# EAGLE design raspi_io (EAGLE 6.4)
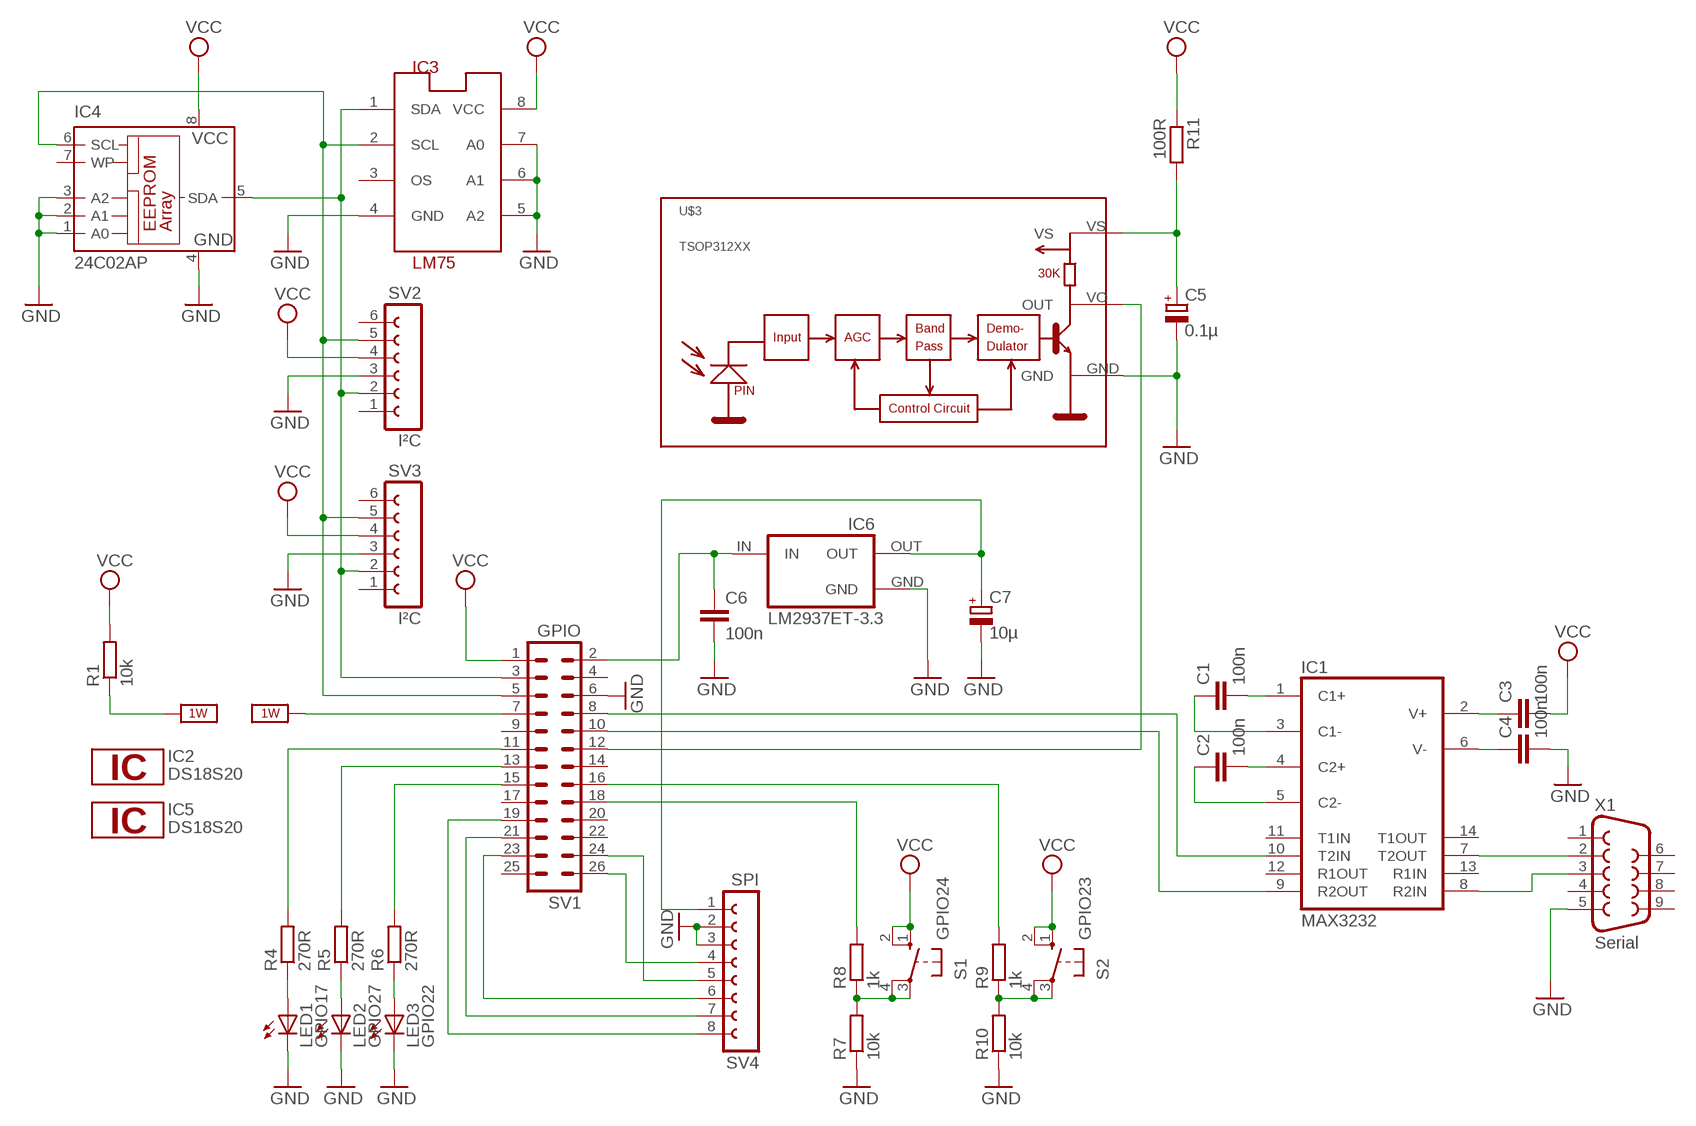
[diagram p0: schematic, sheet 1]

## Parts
C1  100n  C-EU025-025X050  [C025-025X050]
C2  100n  C-EU025-025X050  [C025-025X050]
C3  100n  C-EU025-025X050  [C025-025X050]
C4  100n  C-EU025-025X050  [C025-025X050]
C5  0.1µ  CPOL-EUE2-5  [E2-5]
C6  100n  C-EU025-025X050  [C025-025X050]
C7  10µ  CPOL-EUE2-5  [E2-5]
IC1  MAX3232  MAX232  [DIL16]
IC2  DS18S20  [TO92-]
IC3  LM75  LM75_ICN  [SO8_LM75]
IC4  24C02AP  [DIL8]
IC5  DS18S20  [TO92-]
IC6  LM2937ET-3.3  [TO220(V)]
LED1  GPIO17  LED3MM  [LED3MM]
LED2  GPIO27  LED3MM  [LED3MM]
LED3  GPIO22  LED3MM  [LED3MM]
R1  10k  R-EU_0207/10  [0207/10]
R4  270R  R-EU_0207/10  [0207/10]
R5  270R  R-EU_0207/10  [0207/10]
R6  270R  R-EU_0207/10  [0207/10]
R7  10k  R-EU_0207/10  [0207/10]
R8  1k  R-EU_0207/10  [0207/10]
R9  1k  R-EU_0207/10  [0207/10]
R10  10k  R-EU_0207/10  [0207/10]
R11  100R  R-EU_0207/10  [0207/10]
S1  GPIO24  10-XX  [B3F-10XX]
S2  GPIO23  10-XX  [B3F-10XX]
SV1  GPIO  ML26  [ML26]
SV2  I²C  FE06-1  [FE06]
SV3  I²C  FE06-1  [FE06]
SV4  SPI  FE08-1  [FE08]
U$3  TSOP312XX  [TSOP312]
X1  Serial  F09HP  [F09HP]

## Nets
1W: R1.1 SV1.7 ; supply symbol labelled 1W_SUP
GND: C4.2 C5.- C6.2 C7.- IC3.4(GND) IC3.5(A2) IC3.6(A1) IC3.7(A0) IC4.1(A0) IC4.2(A1) IC4.3(A2) IC4.4(GND) IC6.GND LED1.K(C) LED2.K(C) LED3.K(C) R7.1 R10.1 SV1.6 SV2.3 SV3.3 SV4.2 SV4.3 U$3.GND X1.5
N$1: C1.2 IC1.1(C1+)
N$2: C1.1 IC1.3(C1-)
N$3: C2.2 IC1.4(C2+)
N$4: C2.1 IC1.5(C2-)
N$5: C3.1 IC1.2(V+)
N$6: C4.1 IC1.6(V-)
N$7: IC1.10(T2IN) SV1.8
N$8: IC1.9(R2OUT) SV1.10
N$9: IC1.7(T2OUT) X1.2
N$10: IC1.8(R2IN) X1.3
N$11: IC3.1(SDA) IC4.5(SDA) SV1.3 SV2.2 SV3.2
N$12: IC3.2(SCL) IC4.6(SCL) SV1.5 SV2.5 SV3.5
N$13: LED1.A R4.1
N$14: LED2.A R5.1
N$15: LED3.A R6.1
N$16: R4.2 SV1.11
N$17: R5.2 SV1.13
N$18: R6.2 SV1.15
N$19: R7.2 R8.1 S1.3(P) S1.4(P1)
N$21: R8.2 SV1.18
N$22: R9.2 SV1.16
N$23: C5.+ R11.2 U$3.VS
N$24: SV1.12 U$3.VO(OUT)
N$25: R9.1 R10.2 S2.3(P) S2.4(P1)
N$26: SV1.19 SV4.8
N$27: SV1.21 SV4.7
N$28: SV1.23 SV4.6
N$29: SV1.24 SV4.5
N$30: SV1.26 SV4.4
N$32: C6.1 IC6.IN SV1.2
N$33: C7.+ IC6.OUT SV4.1
VCC: C3.2 IC3.8(VCC) IC4.8(VCC) R1.2 R11.1 S1.1(S) S1.2(S1) S2.1(S) S2.2(S1) SV1.1 SV2.4 SV3.4
Unconnected: IC1.11(T1IN) IC1.12(R1OUT) IC1.13(R1IN) IC1.14(T1OUT) IC3.3(OS) IC4.7(WP) SV1.4 SV1.9 SV1.14 SV1.17 SV1.20 SV1.22 SV1.25 SV2.1 SV2.6 SV3.1 SV3.6 X1.1 X1.4 X1.6 X1.7 X1.8 X1.9

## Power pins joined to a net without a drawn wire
1W: IC2.2 IC5.2
GND: IC1.15(GND) IC2.1 IC5.1
VCC: IC1.16(VCC) IC2.3 IC5.3

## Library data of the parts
C1-C4 C6 = rcl:C-EU: CAPACITOR, European symbol
C5 C7 = rcl:CPOL-EU: POLARIZED CAPACITOR, European symbol
IC1 = maxim:MAX232: RS232 TRANSEIVER; MF: MAXIM; MPN: MAX232ACPE+; OC_FARNELL: 9723773; OC_NEWARK: 68K4544
IC2 IC5 = 1wire:DS18S20: High Precision Digital Thermometer This chip provides a onewire thermosensor with approx. 0.5°C accuracy.A programmable over/undertemperure alarm is available. Notes: Vdd must be applied for accurate measurements at low temperatures, as the parasite power circuit otherwise heats the sensor. If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
IC3 = lm75:LM75_IC: Temperatursensor
IC4 = microchip:24*: Serial EEPROM I2C; MF: MICROCHIP; MPN: 24C02C-I/P; OC_FARNELL: 1755843; OC_NEWARK: 96K4062
IC6 = lm2937:LM2937ET*: 400 and 500 mA Low Dropout Voltage Regulator NATIONAL SEMICONDUCTOR created by Peter.Hofmann@ph-tronic.de 10-2004 Rev.0
LED1-LED3 = led:LED: LED
R1 R4-R11 = rcl:R-EU_: RESISTOR, European symbol
S1 S2 = switch-omron:10-XX: OMRON SWITCH; MPN: B3F-1000; OC_FARNELL: 176432; OC_NEWARK: 36M3542
SV1 = con-harting-ml:ML26: HARTING; OC_FARNELL: unknown; OC_NEWARK: unknown
SV2 SV3 = con-lsta:FE06-1: FEMALE HEADER; OC_FARNELL: unknown; OC_NEWARK: unknown
SV4 = con-lsta:FE08-1: FEMALE HEADER; OC_FARNELL: unknown; OC_NEWARK: unknown
U$3 = vishay:TSOP312XX
X1 = con-subd:F09: SUB-D; OC_FARNELL: unknown; OC_NEWARK: unknown

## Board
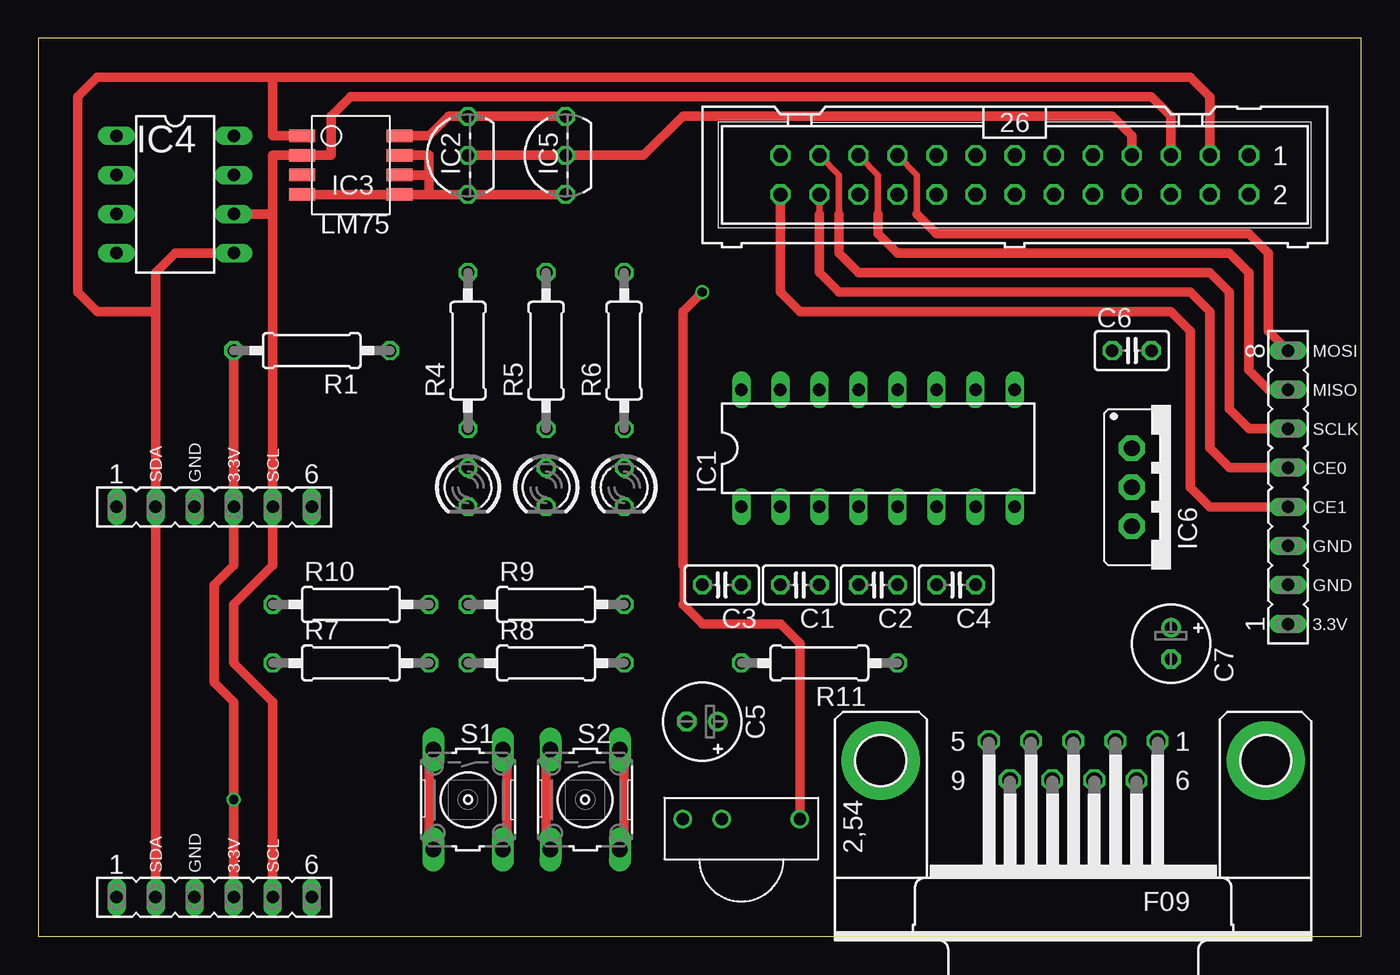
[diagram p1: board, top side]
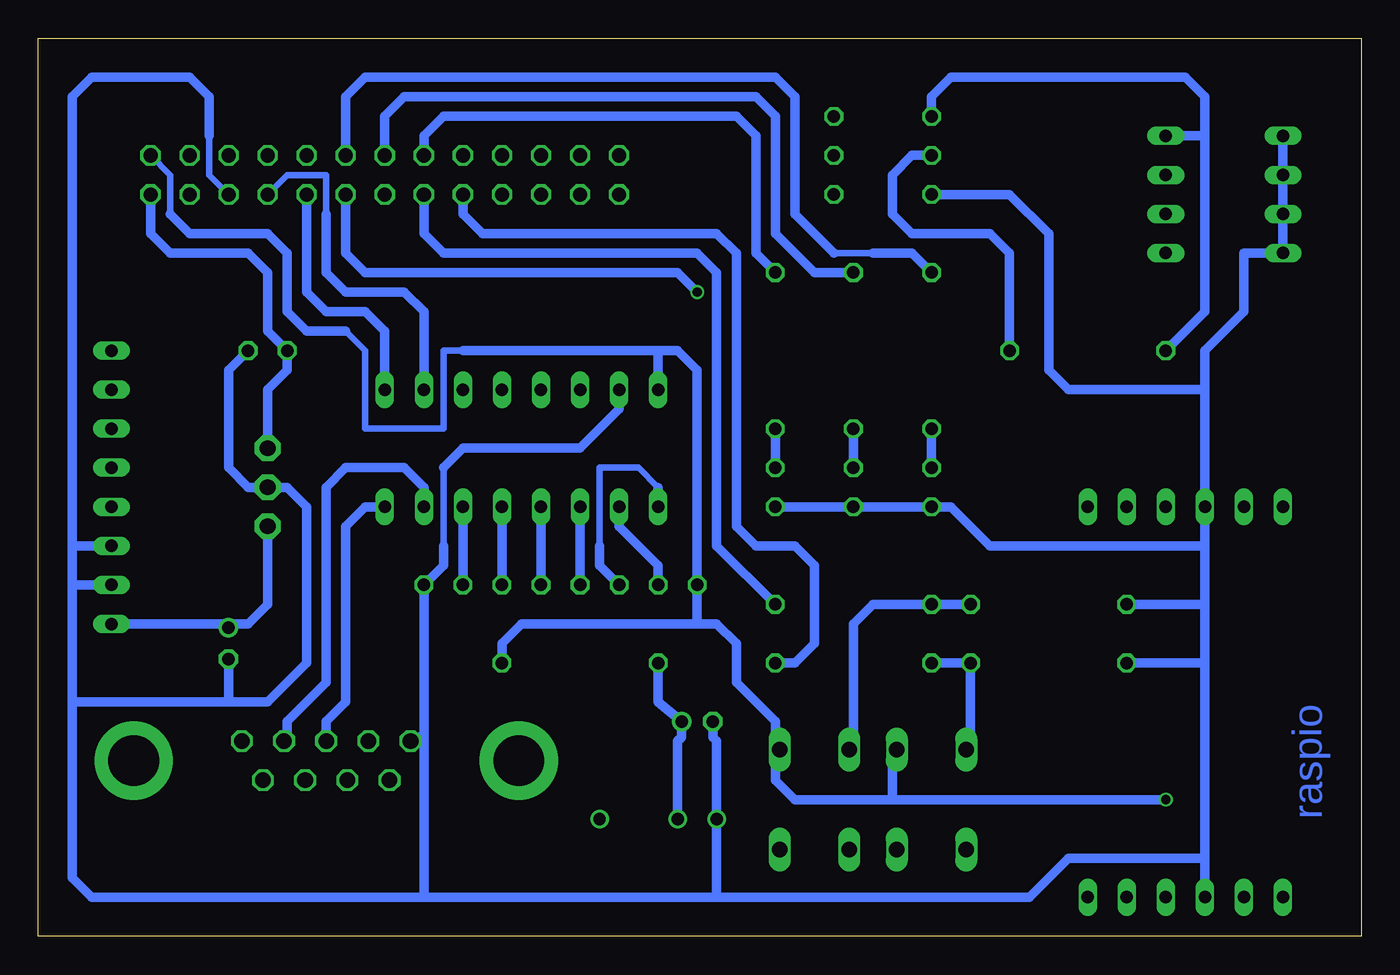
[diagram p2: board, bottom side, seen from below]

Size 86.03 x 58.41 mm. Coordinates in mm from the lower left corner, seen from the top.
Outline: 0,0 86.03,0 86.03,58.41 0,58.41 0,0
Copper layers (1*16): Top 0.035mm / dielectric 1.5mm / Bottom 0.035mm
Design rules "PCB-POOL Standard": minimum track width 0.15mm, minimum drill 0.3mm, track to track 0.15mm, track to pad 0.15mm, pad to pad 0.15mm, via to via 0.15mm, smd to smd 0.15mm, copper to edge 0.3mm, drill to drill 0.2mm, minimum pad ring 0.2mm, minimum via ring 0.15mm, stop-mask expansion 0.075mm, vias tented up to drill 0mil, thermal gap 0.2mm

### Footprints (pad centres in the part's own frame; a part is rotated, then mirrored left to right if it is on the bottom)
C025-025X050 = drill 0.813 octagon: 1 -1.27,0; 2 1.27,0
E2-5 = drill 0.813 pad 1.27: + -1.016,0 | drill 0.813 pad 1.27 octagon: - 1.016,0
DIL16 = drill 0.813 long: 1 -8.89,-3.81; 2 -6.35,-3.81; 3 -3.81,-3.81; 4 -1.27,-3.81; 5 1.27,-3.81; 6 3.81,-3.81; 7 6.35,-3.81; 8 8.89,-3.81; 9 8.89,3.81; 10 6.35,3.81; 11 3.81,3.81; 12 1.27,3.81; 13 -1.27,3.81; 14 -3.81,3.81; 15 -6.35,3.81; 16 -8.89,3.81
TO92- = drill 0.813 octagon: 1 -2.54,0; 2 0,0; 3 2.54,0
SO8_LM75 = smd 0.813 x 1.676: 1 -1.27,-3.175; 2 0,-3.175; 3 1.27,-3.175; 4 2.54,-3.175; 5 2.54,3.175; 6 1.27,3.175; 7 0,3.175; 8 -1.27,3.175
DIL8 = drill 0.813 long: 1 -3.81,-3.81; 2 -1.27,-3.81; 3 1.27,-3.81; 4 3.81,-3.81; 5 3.81,3.81; 6 1.27,3.81; 7 -1.27,3.81; 8 -3.81,3.81
TO220(V) = drill 1.016 pad 1.676 octagon: GND 0,0; IN -2.54,0; OUT 2.54,0
LED3MM = drill 0.813 octagon: A -1.27,0; K 1.27,0
0207/10 = drill 0.813 octagon: 1 -5.08,0; 2 5.08,0
B3F-10XX = drill 1.016 long: 1 -3.251,2.261; 2 3.251,2.261; 3 -3.251,-2.261; 4 3.251,-2.261
ML26 = drill 0.914 octagon: 1 -15.24,-1.27; 2 -15.24,1.27; 3 -12.7,-1.27; 4 -12.7,1.27; 5 -10.16,-1.27; 6 -10.16,1.27; 7 -7.62,-1.27; 8 -7.62,1.27; 9 -5.08,-1.27; 10 -5.08,1.27; 11 -2.54,-1.27; 12 -2.54,1.27; 13 0,-1.27; 14 0,1.27; 15 2.54,-1.27; 16 2.54,1.27; 17 5.08,-1.27; 18 5.08,1.27; 19 7.62,-1.27; 20 7.62,1.27; 21 10.16,-1.27; 22 10.16,1.27; 23 12.7,-1.27; 24 12.7,1.27; 25 15.24,-1.27; 26 15.24,1.27
FE06 = drill 0.813 long: 1 -6.35,0; 2 -3.81,0; 3 -1.27,0; 4 1.27,0; 5 3.81,0; 6 6.35,0
FE08 = drill 0.813 long: 1 -8.89,0; 2 -6.35,0; 3 -3.81,0; 4 -1.27,0; 5 1.27,0; 6 3.81,0; 7 6.35,0; 8 8.89,0
TSOP312 = drill 0.8: GND -3.81,0; VO 3.81,0; VS -1.27,0
F09HP = drill 1.016 octagon: 1 -5.486,-1.27; 2 -2.743,-1.27; 3 0,-1.27; 4 2.743,-1.27; 5 5.486,-1.27; 6 -4.115,1.27; 7 -1.372,1.27; 8 1.372,1.27; 9 4.115,1.27 | drill 3.302 pad 5.08: G1 -12.522,0; G2 12.522,0

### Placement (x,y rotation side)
C1  49.53,22.86 180 top
C2  54.61,22.86 180 top
C3  44.45,22.86 180 top
C4  59.69,22.86 0 top
C5  43.18,13.97 180 top
C6  71.12,38.1 0 top
C7  73.66,19.05 270 top
IC1  54.61,31.75 0 top
IC2  27.94,50.8 90 top
IC3  20.32,50.8 270 top
IC4  8.89,48.26 270 top
IC5  34.29,50.8 90 top
IC6  71.12,29.21 270 top
LED1  27.94,29.21 270 top
LED2  33.02,29.21 270 top
LED3  38.1,29.21 270 top
R1  17.78,38.1 180 top
R4  27.94,38.1 90 top
R5  33.02,38.1 90 top
R6  38.1,38.1 90 top
R7  20.32,17.78 0 top
R8  33.02,17.78 0 top
R9  33.02,21.59 0 top
R10  20.32,21.59 0 top
R11  50.8,17.78 180 top
S1  27.94,8.89 270 top
S2  35.56,8.89 270 top
SV1  63.5,49.53 180 top
SV2  11.43,27.94 0 top
SV3  11.43,2.54 0 top
SV4  81.28,29.21 90 top
U$3  45.72,7.62 0 top
X1  67.31,11.43 180 top

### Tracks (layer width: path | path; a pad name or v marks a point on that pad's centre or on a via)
1W
  Top 0.61: IC2.2 IC5.2 39.37,50.8 41.91,53.34 69.85,53.34 71.12,52.07 SV1.7
  Bottom 0.61: IC2.2 29.21,50.8 30.48,49.53 30.48,46.99 29.21,45.72 24.13,45.72 22.86,44.45 R1.1
GND
  Top 0.61: IC3.7 25.4,50.8 25.4,49.53 | 25.4,49.53 25.4,48.26 | 25.4,48.26 IC2.1 IC5.1 | IC3.4 IC3.5 25.4,48.26 | IC3.6 25.4,49.53
  Bottom 0.406: SV1.6 74.93,49.53 74.93,52.07 | 59.69,30.48 59.69,25.4
  Bottom 0.61: LED3.K LED2.K LED1.K 26.67,27.94 24.13,25.4 10.16,25.4 | IC4.1 IC4.2 IC4.3 IC4.4 7.62,44.45 7.62,40.64 10.16,38.1 10.16,35.56 | 74.93,52.07 74.93,54.61 76.2,55.88 82.55,55.88 83.82,54.61 83.82,25.4 | 83.82,25.4 83.82,22.86 | 83.82,22.86 83.82,15.24 | 83.82,15.24 83.82,3.81 82.55,2.54 60.96,2.54 | 60.96,2.54 60.96,13.11 | 41.91,2.54 60.96,2.54 | 41.91,2.54 U$3.GND 41.91,12.7 42.16,12.95 C5.- | 41.91,2.54 21.59,2.54 19.05,5.08 10.16,5.08 | 12.7,17.78 R7.1 10.16,17.78 | 60.96,13.11 C4.2 59.69,24.13 59.69,25.4 | 60.96,13.11 X1.5 | IC1.15 48.26,34.29 50.8,31.75 58.42,31.75 59.69,30.48 | 73.66,15.24 71.12,15.24 68.58,17.78 68.58,27.94 69.85,29.21 IC6.GND 72.39,29.21 73.66,30.48 73.66,36.83 C6.2 | 73.66,15.24 83.82,15.24 | SV4.2 83.82,22.86 | SV4.3 83.82,25.4 | C7.- 73.66,15.24 | 10.16,35.56 SV2.3 10.16,25.4 | 10.16,25.4 10.16,21.59 | 10.16,21.59 10.16,17.78 | 10.16,17.78 10.16,5.08 | 10.16,5.08 SV3.3 | R10.1 10.16,21.59 | 10.16,35.56 19.05,35.56 20.32,36.83 20.32,45.72 22.86,48.26 IC2.1
N$1
  Bottom 0.406: 45.72,29.21 46.99,30.48 49.53,30.48 49.53,25.4
  Bottom 0.61: IC1.1 45.72,29.21 | 49.53,25.4 49.53,24.13 C1.2
N$2
  Bottom 0.61: IC1.3 C1.1
N$3
  Bottom 0.61: IC1.4 C2.2
N$4
  Bottom 0.61: IC1.5 C2.1
N$5
  Bottom 0.61: IC1.2 48.26,26.67 45.72,24.13 C3.1
N$6
  Bottom 0.61: IC1.6 C4.1
N$7
  Bottom 0.406: SV1.8 69.85,49.53 67.31,49.53 67.31,46.99
  Bottom 0.61: 67.31,46.99 67.31,43.18 66.04,41.91 62.23,41.91 60.96,40.64 IC1.10
N$8
  Bottom 0.61: SV1.10 68.58,41.91 67.31,40.64 64.77,40.64 63.5,39.37 IC1.9
N$9
  Bottom 0.61: IC1.7 60.96,29.21 62.23,30.48 66.04,30.48 67.31,29.21 67.31,16.51 69.85,13.97 69.85,12.9 X1.2
N$10
  Bottom 0.61: IC1.8 64.77,27.94 66.04,26.67 66.04,15.24 67.31,13.97 X1.3
N$11
  Top 0.61: SV1.3 76.2,54.61 74.93,55.88 15.24,55.88 | 15.24,55.88 3.81,55.88 2.54,54.61 2.54,41.91 3.81,40.64 7.62,40.64 | SV3.2 SV2.2 7.62,40.64 | IC3.1 15.24,52.07 15.24,55.88 | IC4.5 8.89,44.45 7.62,43.18 7.62,40.64
N$12
  Top 0.61: SV1.5 73.66,53.34 72.39,54.61 20.32,54.61 19.05,53.34 19.05,50.8 IC3.2 15.24,50.8 15.24,46.99 | SV3.5 15.24,15.24 12.7,17.78 12.7,21.59 15.24,24.13 SV2.5 15.24,46.99 | IC4.6 15.24,46.99
N$13
  Bottom 0.61: R4.1 LED1.A
N$14
  Bottom 0.61: R5.1 LED2.A
N$15
  Bottom 0.61: R6.1 LED3.A
N$16
  Bottom 0.406: 31.75,44.45 34.29,44.45
  Bottom 0.61: R4.2 29.21,44.45 31.75,44.45 | 34.29,44.45 36.83,46.99 36.83,54.61 38.1,55.88 64.77,55.88 66.04,54.61 SV1.11
N$17
  Bottom 0.61: R5.2 35.56,43.18 38.1,45.72 38.1,53.34 39.37,54.61 62.23,54.61 63.5,53.34 SV1.13
N$18
  Bottom 0.61: R6.2 39.37,44.45 39.37,52.07 40.64,53.34 59.69,53.34 60.96,52.07 SV1.15
N$19
  Top 0.61: S1.3 25.68,11.71 25.4,11.43 25.4,5.92 S1.4
  Bottom 0.61: R8.1 R7.2 25.4,12.42 S1.3
N$21
  Bottom 0.61: SV1.18 58.42,46.99 57.15,45.72 41.91,45.72 40.64,44.45 40.64,26.67 39.37,25.4 36.83,25.4 35.56,24.13 35.56,19.05 36.83,17.78 R8.2
N$22
  Bottom 0.61: SV1.16 60.96,45.72 59.69,44.45 43.18,44.45 41.91,43.18 41.91,25.4 R9.2
N$23
  Bottom 0.61: R11.2 45.72,15.24 C5.+ 44.2,12.95 44.45,12.7 U$3.VS
N$24  (via drill 0.6)
  Top 0.406: 41.91,24.13 41.91,21.59
  Top 0.61: v43.18,41.91 41.91,40.64 41.91,24.13 | 41.91,21.59 43.18,20.32 48.26,20.32 49.53,19.05 U$3.VO
  Bottom 0.61: SV1.12 66.04,44.45 64.77,43.18 44.45,43.18 v43.18,41.91
N$25
  Top 0.61: S2.3 33.3,11.71 33.02,11.43 33.02,5.92 S2.4
  Bottom 0.61: R9.1 R10.2 31.75,21.59 33.02,20.32 33.02,12.42 S2.3
N$26
  Top 0.406: SV1.19 57.15,49.53 57.15,46.99
  Top 0.61: 57.15,46.99 58.42,45.72 78.74,45.72 80.01,44.45 80.01,39.37 SV4.8
N$27
  Top 0.406: SV1.21 54.61,49.53 54.61,46.99
  Top 0.61: 54.61,46.99 54.61,45.72 55.88,44.45 77.47,44.45 78.74,43.18 78.74,36.83 80.01,35.56 SV4.7
N$28
  Top 0.406: SV1.23 52.07,49.53 52.07,46.99
  Top 0.61: 52.07,46.99 52.07,44.45 53.34,43.18 76.2,43.18 77.47,41.91 77.47,34.29 78.74,33.02 SV4.6
N$29
  Top 0.406: SV1.24 50.8,46.99
  Top 0.61: 50.8,46.99 50.8,43.18 52.07,41.91 74.93,41.91 76.2,40.64 76.2,31.75 77.47,30.48 SV4.5
N$30
  Top 0.61: SV1.26 48.26,41.91 49.53,40.64 73.66,40.64 74.93,39.37 74.93,29.21 76.2,27.94 SV4.4
N$32
  Bottom 0.61: SV1.2 78.74,45.72 77.47,44.45 72.39,44.45 71.12,43.18 71.12,39.37 C6.1 69.85,36.83 71.12,35.56 IC6.IN
N$33
  Bottom 0.61: IC6.OUT 71.12,21.59 72.39,20.32 73.66,20.32 | 73.66,20.32 SV4.1 | C7.+ 73.66,20.32
VCC  (via drill 0.6)
  Top 0.61: IC3.8 25.4,52.07 26.67,53.34 IC2.3 IC5.3 | S1.2 30.2,6.07 30.48,6.35 30.48,11.86 S1.1 | S2.2 37.82,6.07 38.1,6.35 38.1,11.86 S2.1 | SV3.4 v12.7,8.89 12.7,15.24 11.43,16.51 11.43,22.86 12.7,24.13 SV2.4 R1.2
  Bottom 0.406: 66.04,39.37 64.77,38.1 64.77,33.02 59.69,33.02 59.69,38.1 58.42,38.1 | SV1.1 77.47,49.53 77.47,46.99
  Bottom 0.61: 66.04,39.37 68.58,39.37 69.85,40.64 69.85,44.45 71.12,45.72 76.2,45.72 77.47,46.99 | 58.42,38.1 45.72,38.1 | IC1.16 45.72,38.1 | 45.72,38.1 44.45,38.1 43.18,36.83 C3.2 43.18,20.32 | IC2.3 27.94,54.61 26.67,55.88 11.43,55.88 10.16,54.61 10.16,52.07 | 43.18,20.32 41.91,20.32 40.64,19.05 40.64,16.51 38.1,13.97 38.1,12.42 S2.1 37.82,11.71 38.1,11.43 38.1,10.16 36.83,8.89 30.48,8.89 | 43.18,20.32 54.61,20.32 55.88,19.05 R11.1 | S1.1 30.2,11.71 30.48,11.43 30.48,8.89 | 10.16,52.07 IC4.8 | 10.16,52.07 10.16,40.64 R1.2 | v12.7,8.89 30.48,8.89

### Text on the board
Bottom: raspio
tNames: MOSI | MISO | SCLK | SDA | GND | 3.3V | SCL | CE0 | CE1 | GND | GND | 3.3V | SDA | GND | 3.3V | SCL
